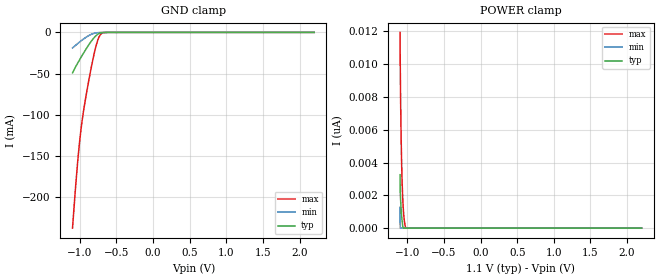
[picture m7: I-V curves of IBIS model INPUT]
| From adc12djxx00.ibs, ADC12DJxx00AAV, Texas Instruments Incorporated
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|   Model INPUT
[Model]   INPUT
Model_type   Input
Vinl = .57
Vinh = 1.33
|   (nom PVT)   (fast PVT)   (slow PVT)
|   typ   min   max
C_comp   0.466p   0.345p   0.547p
[Voltage Range]   1.1   1.05   1.15
[Temperature Range]   27   125   -40
[Power Clamp Reference]   1.1   1.05   1.15
[GND Clamp Reference]   0   0   0
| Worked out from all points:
|   GND clamp passes 1 mA (typ) near -0.72 V on its own axis
[GND Clamp]
|   Voltage   I(typ)   I(min)   I(max)
-1.1V     -49.14mA   -18.92mA   -237.6mA
-1.06V    -42.27mA   -15.9mA    -190.3mA
-1.024V   -36.47mA   -13.22mA   -151.7mA
-1.004V   -33.4mA    -11.79mA   -133.5mA
-987.8mV  -30.88mA   -10.63mA   -120.3mA
-951.5mV  -25.45mA   -8.189mA   -96.5mA
-882.2mV  -15.65mA   -4.119mA   -60.46mA
-799.7mV  -5.845mA   -1.039mA   -23.94mA
-750.2mV  -2.053mA   -317.8uA   -8.184mA
-704mV    -501uA     -91.38uA   -1.518mA
-618.2mV  -21.62uA   -8.11uA    -26.33uA
2.2V      0A         0A         0A
[POWER Clamp]
|   Voltage   I(typ)   I(min)   I(max)
-1.1V     3.257nA    1.268nA    11.94nA
-1.097V   2.17nA     0A         9.854nA
-1.093V   1.84nA     0A         8.403nA
-1.087V   1.291nA    0A         6.094nA
-1.08V    862.3pA    0A         4.397nA
-1.077V   683.9pA    0A         3.726nA
-1.07V    388pA      0A         2.658nA
-1.06V    60.49pA    0A         1.562nA
-1.047V   0A         0A         703.5pA
-1.031V   0A         0A         161.3pA
-1.018V   0A         0A         0A
2.2V      0A         0A         0A
